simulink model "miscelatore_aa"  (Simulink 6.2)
settings: Solver=ode45  StartTime=0.0  StopTime=1000  RelTol=1e-3
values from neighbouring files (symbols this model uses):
  A = pi    (= 3.14159265359)    [dati_miscelatore.m]
  c = 4200    [dati_miscelatore.m]
  k = 0.36    [dati_miscelatore.m]
  R = ((c*w1+c*w2+k*A)*T-c*w1*T1-c*w2*T2-k*A*Ta)/(i^2)    (= 7560)    [dati_miscelatore.m]
  rho = 1000    [dati_miscelatore.m]
  T1 = 273+50    (= 323)    [dati_miscelatore.m]
  T2 = 273+10    (= 283)    [dati_miscelatore.m]
  Ta = 273+20    (= 293)    [dati_miscelatore.m]
undefined symbols (not defined in the file or in its folder): miscelatore

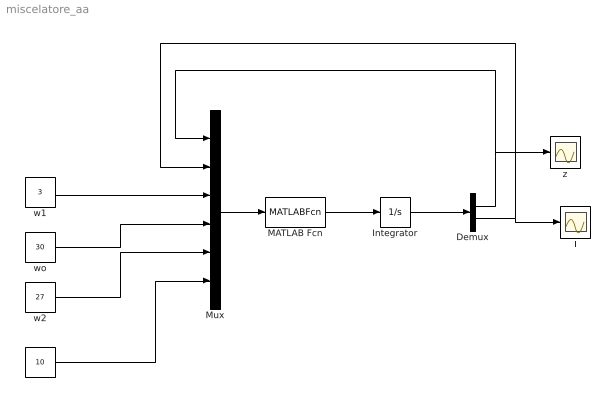
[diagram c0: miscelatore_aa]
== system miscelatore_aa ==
  Demux : Demux  Outputs=2
  Integrator : Integrator  InitialCondition=[1 273+20]
  MATLAB Fcn : MATLABFcn  MATLABFcn=miscelatore(u,rho,A,c,T1,T2,Ta,k,R)  OutputDimensions=2
  Mux : Mux  Inputs=6
  T : Scope
  i : Constant  Value=10
  w1 : Constant  Value=3
  w2 : Constant  Value=27
  wo : Constant  Value=30
  z : Scope
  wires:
  Mux/1 -> MATLAB Fcn/1
  Demux/1 -> Mux/1, z/1
  Demux/2 -> Mux/2, T/1
  w1/1 -> Mux/3
  wo/1 -> Mux/4
  w2/1 -> Mux/5
  i/1 -> Mux/6
  MATLAB Fcn/1 -> Integrator/1
  Integrator/1 -> Demux/1
